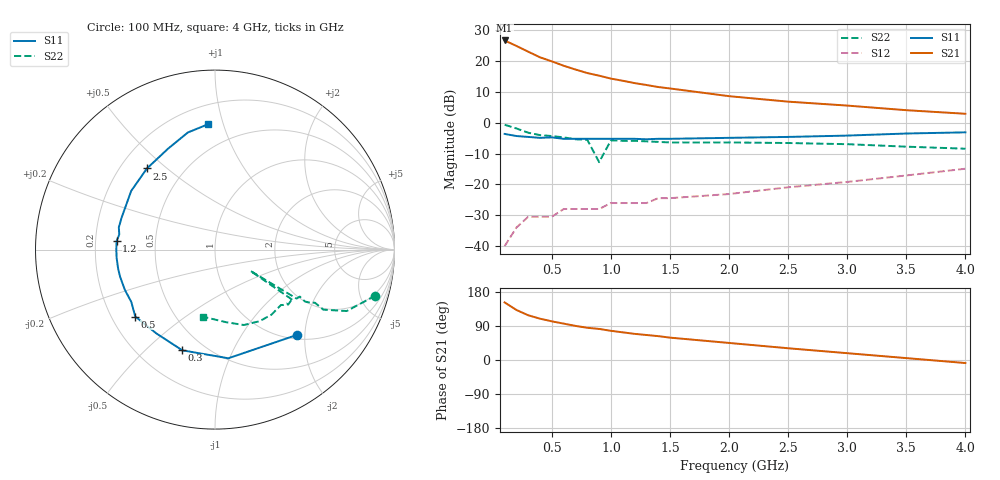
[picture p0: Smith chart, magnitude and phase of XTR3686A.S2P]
! HXTR-3686 Typical S-Parameters
!  (Vce =10 V, Ic = 10 mA)
# ghz s ma r 50
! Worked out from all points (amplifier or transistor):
!   20 points, 100 MHz to 4 GHz, reference 50 ohm
!   highest |S21| = 26.7 dB at 100 MHz (marker M1)
!   |S21| within 3 dB of that: start of sweep to 265.5 MHz
!   unconditionally stable (mu >= 1): 815.3 MHz to 983.3 MHz; 1.175 GHz to 3.064 GHz
!   at 400 MHz: K = 0.55, MSG = 25.8 dB, |S12| = -30.5 dB
!   at 1.1 GHz: K = 0.94, MSG = 19.8 dB, |S12| = -26.0 dB
!   at 4 GHz: K = 0.78, MSG = 8.9 dB, |S12| = -14.9 dB
!   S11 on the Smith chart (normalised r, x): 100 MHz: 1.09, -1.83; 300 MHz: 0.38, -0.66; 500 MHz: 0.30, -0.34; 1.2 GHz: 0.29, +0.04; 2.5 GHz: 0.31, +0.43; 4 GHz: 0.33, +0.89
0.1  0.66 -46.0  21.6 152.0  0.01 68.0  0.93 -16.0
0.2  0.61 -83.0  17.6 132.0  0.02 55.0  0.81 -25.0
0.3  0.59 -108.0  14.2 118.0  0.03 48.0  0.69 -29.0
0.4  0.57 -125.0  11.5 109.0  0.03 45.0  0.63 -28.0
0.5  0.58 -140.0  9.9 102.0  0.03 43.0  0.61 -29.0
0.6  0.55 -148.0  8.4 96.0  0.04 44.0  0.58 -30.0
0.7  0.55 -156.0  7.3 90.0  0.04 44.0  0.54 -29.0
0.8  0.55 -164.0  6.4 85.0  0.04 45.0  0.53 -31.0
0.9  0.55 -169.0  5.8 82.0  0.04 46.0  0.23 -31.0
1  0.55 -175.0  5.2 77.0  0.05 47.0  0.52 -33.0
1.1  0.55 180.0  4.8 73.0  0.05 48.0  0.51 -34.0
1.2  0.55 175.0  4.4 69.0  0.05 48.0  0.51 -37.0
1.3  0.54 171.0  4.1 66.0  0.05 49.0  0.5 -37.0
1.4  0.55 167.0  3.8 63.0  0.06 50.0  0.49 -39.0
1.5  0.55 161.0  3.6 59.0  0.06 51.0  0.48 -40.0
2  0.57 145.0  2.7 45.0  0.07 52.0  0.48 -49.0
2.5  0.59 130.0  2.2 31.0  0.09 51.0  0.47 -58.0
3  0.62 115.0  1.9 18.0  0.11 49.0  0.45 -69.0
3.5  0.67 103.0  1.6 5.0  0.14 44.0  0.41 -81.0
4  0.7 93.0  1.4 -8.0  0.18 37.0  0.38 -100.0
